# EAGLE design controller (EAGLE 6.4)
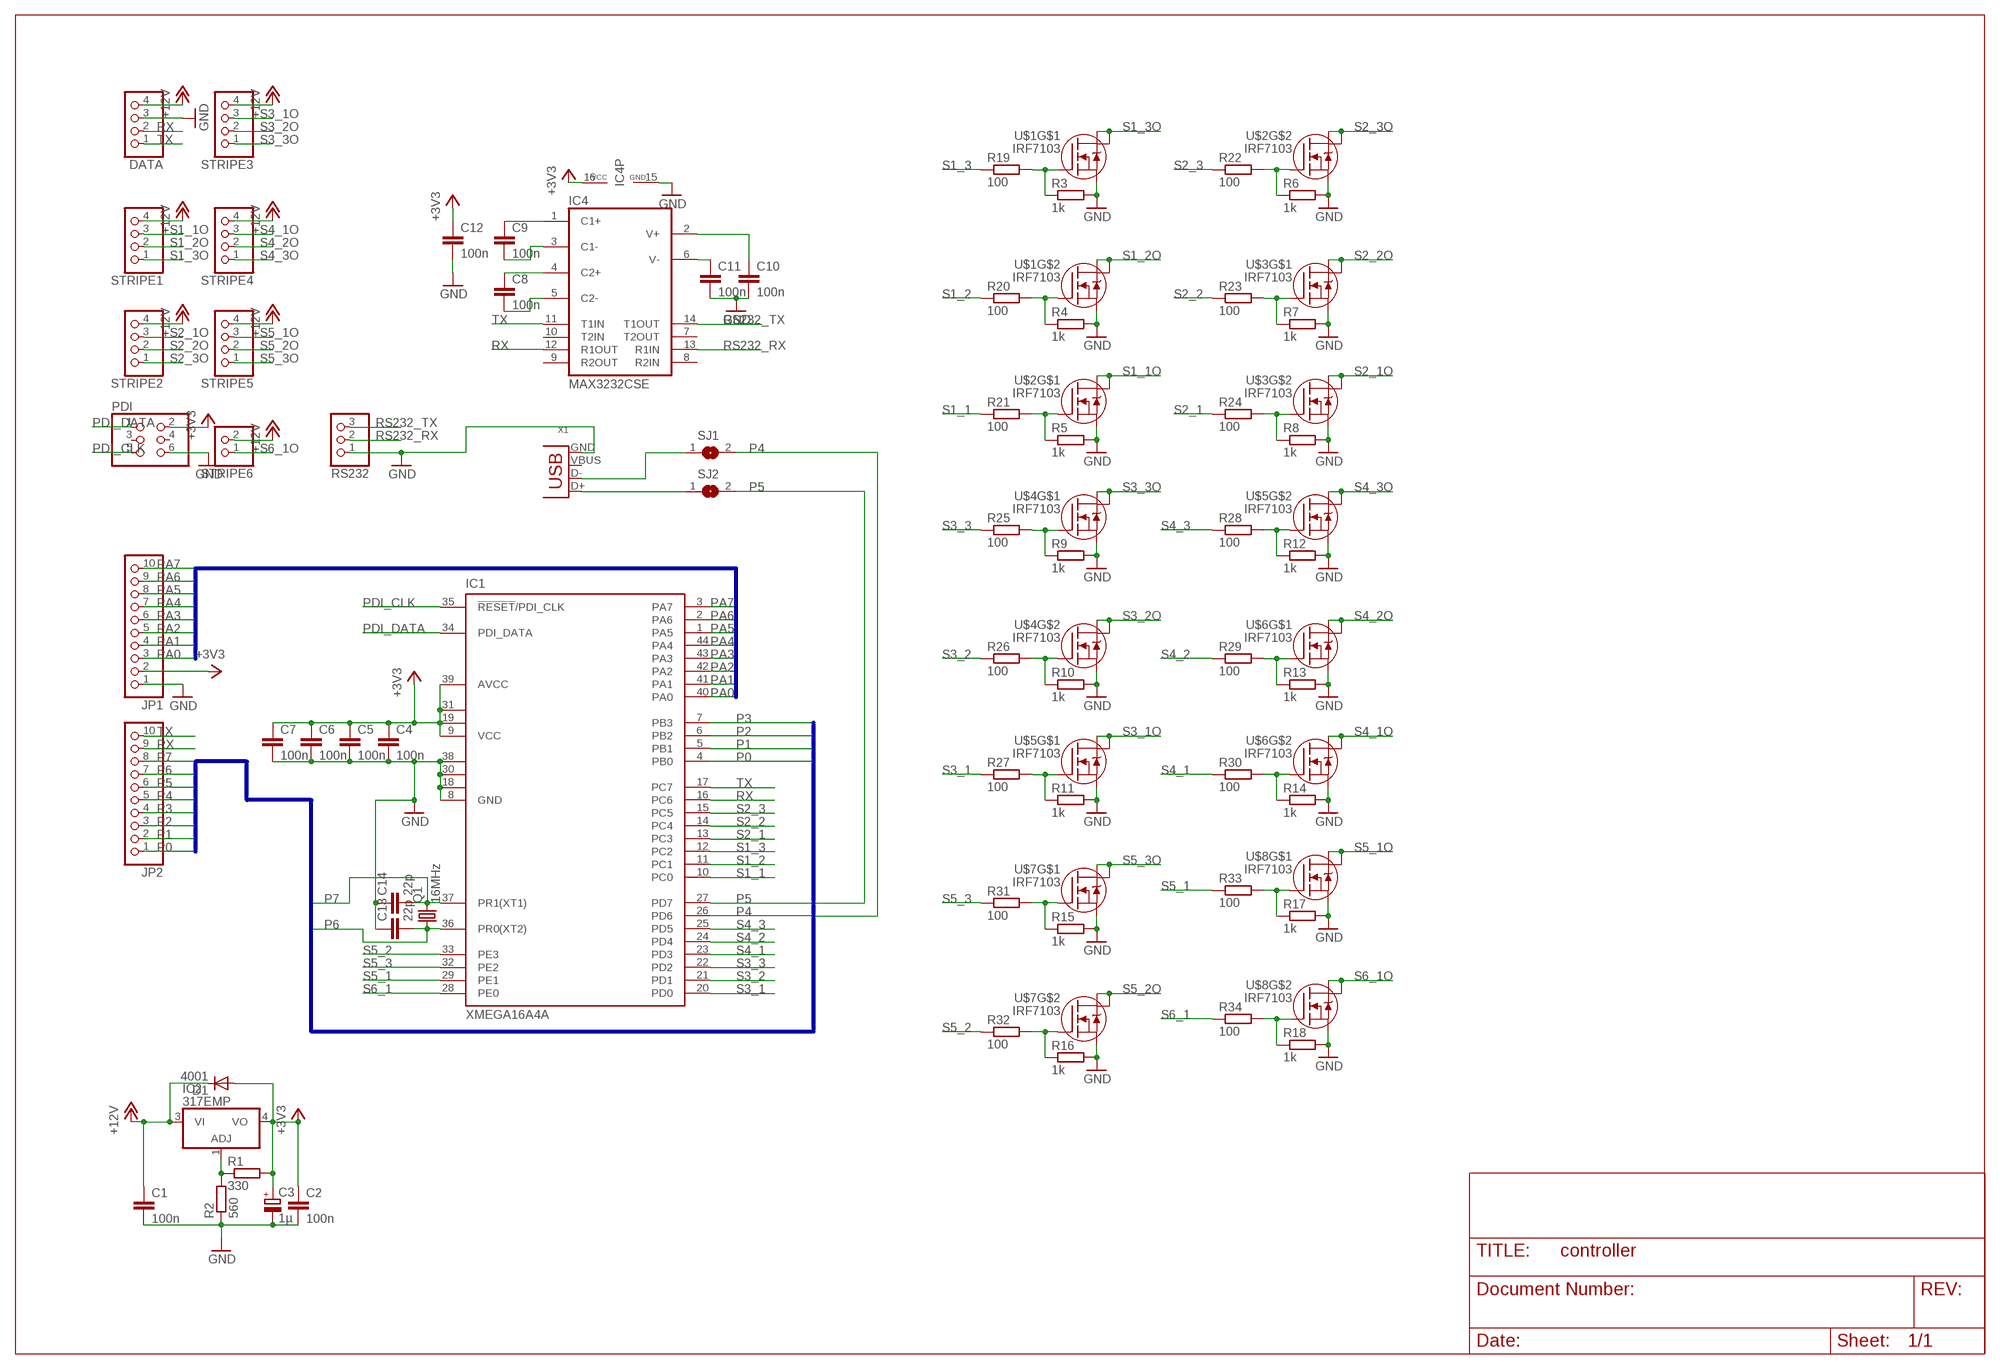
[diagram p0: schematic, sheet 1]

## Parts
C1  100n  C-EUC0805K  [C0805K]
C2  100n  C-EUC0805K  [C0805K]
C3  1µ  CPOL-EUSMCB  [SMC_B]
C4  100n  C-EUC0805K  [C0805K]
C5  100n  C-EUC0805K  [C0805K]
C6  100n  C-EUC0805K  [C0805K]
C7  100n  C-EUC0805K  [C0805K]
C8  100n  C-EUC0805K  [C0805K]
C9  100n  C-EUC0805K  [C0805K]
C10  100n  C-EUC0805K  [C0805K]
C11  100n  C-EUC0805K  [C0805K]
C12  100n  C-EUC0805K  [C0805K]
C13  22p  C-EUC0805K  [C0805K]
C14  22p  C-EUC0805K  [C0805K]
D1  4001  DIODE-MELF-MLL41  [MELF-MLL41]
DATA  PINHD-1X4  [1X04]
IC1  XMEGA16A4A  [TQFP44]
IC2  317EMP  [SOT223]
IC4  MAX3232CSE  [SO16]
JP1  PINHD-1X10  [1X10]
JP2  PINHD-1X10  [1X10]
PDI  PINHD-2X3  [2X03]
Q1  16MHz  CRYSTALHC49S  [HC49/S]
R1  330  R-EU_R0603  [R0603]
R2  560  R-EU_R0603  [R0603]
R3  1k  R-EU_R0603  [R0603]
R4  1k  R-EU_R0603  [R0603]
R5  1k  R-EU_R0603  [R0603]
R6  1k  R-EU_R0603  [R0603]
R7  1k  R-EU_R0603  [R0603]
R8  1k  R-EU_R0603  [R0603]
R9  1k  R-EU_R0603  [R0603]
R10  1k  R-EU_R0603  [R0603]
R11  1k  R-EU_R0603  [R0603]
R12  1k  R-EU_R0603  [R0603]
R13  1k  R-EU_R0603  [R0603]
R14  1k  R-EU_R0603  [R0603]
R15  1k  R-EU_R0603  [R0603]
R16  1k  R-EU_R0603  [R0603]
R17  1k  R-EU_R0603  [R0603]
R18  1k  R-EU_R0603  [R0603]
R19  100  R-EU_R0603  [R0603]
R20  100  R-EU_R0603  [R0603]
R21  100  R-EU_R0603  [R0603]
R22  100  R-EU_R0603  [R0603]
R23  100  R-EU_R0603  [R0603]
R24  100  R-EU_R0603  [R0603]
R25  100  R-EU_R0603  [R0603]
R26  100  R-EU_R0603  [R0603]
R27  100  R-EU_R0603  [R0603]
R28  100  R-EU_R0603  [R0603]
R29  100  R-EU_R0603  [R0603]
R30  100  R-EU_R0603  [R0603]
R31  100  R-EU_R0603  [R0603]
R32  100  R-EU_R0603  [R0603]
R33  100  R-EU_R0603  [R0603]
R34  100  R-EU_R0603  [R0603]
RS232  PINHD-1X3  [1X03]
SJ1  SJ  [SJ]
SJ2  SJ  [SJ]
STRIPE1  PINHD-1X4  [1X04]
STRIPE2  PINHD-1X4  [1X04]
STRIPE3  PINHD-1X4  [1X04]
STRIPE4  PINHD-1X4  [1X04]
STRIPE5  PINHD-1X4  [1X04]
STRIPE6  PINHD-1X2  [1X02]
U$1  IRF7103  [SO8-2]
U$2  IRF7103  [SO8-2]
U$3  IRF7103  [SO8-2]
U$4  IRF7103  [SO8-2]
U$5  IRF7103  [SO8-2]
U$6  IRF7103  [SO8-2]
U$7  IRF7103  [SO8-2]
U$8  IRF7103  [SO8-2]
X1  USB-MB-H  [USB-MB-H]

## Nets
+3V3: C2.1 C3.+ C4.1 C5.1 C6.1 C7.1 C12.1 D1.A IC1.9(VCC) IC1.19(VCC1) IC1.31(VCC2) IC1.39(AVCC) IC2.4(VO) IC4.16(VCC) JP1.2 PDI.2 R1.2
+12V: C1.1 D1.C DATA.4 IC2.3(VI) STRIPE1.4 STRIPE2.4 STRIPE3.4 STRIPE4.4 STRIPE5.4 STRIPE6.2
GND: C1.2 C2.2 C3.- C4.2 C5.2 C6.2 C7.2 C10.2 C11.2 C12.2 C13.1 C14.1 DATA.3 IC1.8(GND) IC1.18(GND1) IC1.30(GND2) IC1.38(GND3) IC4.15(GND) JP1.1 PDI.6 R2.1 R3.2 R4.2 R5.2 R6.2 R7.2 R8.2 R9.2 R10.2 R11.2 R12.2 R13.2 R14.2 R15.2 R16.2 R17.2 R18.2 RS232.1 U$1.1(S) U$1.3(S) U$2.1(S) U$2.3(S) U$3.1(S) U$3.3(S) U$4.1(S) U$4.3(S) U$5.1(S) U$5.3(S) U$6.1(S) U$6.3(S) U$7.1(S) U$7.3(S) U$8.1(S) U$8.3(S) X1.GND
N$1: C8.1 IC4.4(C2+)
N$2: C8.2 IC4.5(C2-)
N$3: C9.1 IC4.1(C1+)
N$4: IC2.1(ADJ) R1.1 R2.2
N$5: C9.2 IC4.3(C1-)
N$6: C10.1 IC4.2(V+)
N$7: C11.1 IC4.6(V-)
N$8: R3.1 R19.2 U$1.2(G)
N$9: R4.1 R20.2 U$1.4(G)
N$10: R5.1 R21.2 U$2.2(G)
N$11: R6.1 R22.2 U$2.4(G)
N$12: R8.1 R24.2 U$3.4(G)
N$13: R11.1 R27.2 U$5.2(G)
N$14: R7.1 R23.2 U$3.2(G)
N$15: R12.1 R28.2 U$5.4(G)
N$16: R9.1 R25.2 U$4.2(G)
N$17: R10.1 R26.2 U$4.4(G)
N$18: R14.1 R30.2 U$6.4(G)
N$19: R15.1 R31.2 U$7.2(G)
N$20: R13.1 R29.2 U$6.2(G)
N$21: R18.1 R34.2 U$8.4(G)
N$22: R16.1 R32.2 U$7.4(G)
N$23: SJ2.1 X1.D+
N$24: R17.1 R33.2 U$8.2(G)
N$25: SJ1.1 X1.D-
P0: IC1.4(PB0) JP2.1
P1: IC1.5(PB1) JP2.2
P2: IC1.6(PB2) JP2.3
P3: IC1.7(PB3) JP2.4
P4: IC1.26(PD6) JP2.5 SJ1.2
P5: IC1.27(PD7) JP2.6 SJ2.2
P6: C13.2 IC1.36(PR0(XT2)) JP2.7 Q1.1
P7: C14.2 IC1.37(PR1(XT1)) JP2.8 Q1.2
PA0: IC1.40(PA0) JP1.3
PA1: IC1.41(PA1) JP1.4
PA2: IC1.42(PA2) JP1.5
PA3: IC1.43(PA3) JP1.6
PA4: IC1.44(PA4) JP1.7
PA5: IC1.1(PA5) JP1.8
PA6: IC1.2(PA6) JP1.9
PA7: IC1.3(PA7) JP1.10
PDI_CLK: IC1.35(!RESET!/PDI_CLK) PDI.5
PDI_DATA: IC1.34(PDI_DATA) PDI.1
RS232_RX: IC4.13(R1IN) RS232.2
RS232_TX: IC4.14(T1OUT) RS232.3
RX: DATA.2 IC1.16(PC6) IC4.12(R1OUT) JP2.9
S1_1: IC1.10(PC0) R21.1
S1_1O: STRIPE1.3 U$2.7(D) U$2.8(D)
S1_2: IC1.11(PC1) R20.1
S1_2O: STRIPE1.2 U$1.5(D) U$1.6(D)
S1_3: IC1.12(PC2) R19.1
S1_3O: STRIPE1.1 U$1.7(D) U$1.8(D)
S2_1: IC1.13(PC3) R24.1
S2_1O: STRIPE2.3 U$3.5(D) U$3.6(D)
S2_2: IC1.14(PC4) R23.1
S2_2O: STRIPE2.2 U$3.7(D) U$3.8(D)
S2_3: IC1.15(PC5) R22.1
S2_3O: STRIPE2.1 U$2.5(D) U$2.6(D)
S3_1: IC1.20(PD0) R27.1
S3_1O: STRIPE3.3 U$5.7(D) U$5.8(D)
S3_2: IC1.21(PD1) R26.1
S3_2O: STRIPE3.2 U$4.5(D) U$4.6(D)
S3_3: IC1.22(PD2) R25.1
S3_3O: STRIPE3.1 U$4.7(D) U$4.8(D)
S4_1: IC1.23(PD3) R30.1
S4_1O: STRIPE4.3 U$6.5(D) U$6.6(D)
S4_2: IC1.24(PD4) R29.1
S4_2O: STRIPE4.2 U$6.7(D) U$6.8(D)
S4_3: IC1.25(PD5) R28.1
S4_3O: STRIPE4.1 U$5.5(D) U$5.6(D)
S5_1: IC1.29(PE1) R33.1
S5_1O: STRIPE5.3 U$8.7(D) U$8.8(D)
S5_2: IC1.33(PE3) R32.1
S5_2O: STRIPE5.2 U$7.5(D) U$7.6(D)
S5_3: IC1.32(PE2) R31.1
S5_3O: STRIPE5.1 U$7.7(D) U$7.8(D)
S6_1: IC1.28(PE0) R34.1
S6_1O: STRIPE6.1 U$8.5(D) U$8.6(D)
TX: DATA.1 IC1.17(PC7) IC4.11(T1IN) JP2.10
Unconnected: IC4.7(T2OUT) IC4.8(R2IN) IC4.9(R2OUT) IC4.10(T2IN) PDI.3 PDI.4 X1.VBUS

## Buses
EXP1:PA[0..7]
EXP2:P[0..7]

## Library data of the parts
C1 C2 C4-C14 = resistor:C-EU: CAPACITOR, European symbol
C3 = resistor:CPOL-EU: POLARIZED CAPACITOR, European symbol
D1 = diode:DIODE-: DIODE
DATA STRIPE1-STRIPE5 = pinhead:PINHD-1X4: PIN HEADER
IC1 = atmel:XMEGA16A4: MICROCONTROLLER Features High-performance, Low-power 8/16-bit AVR XMEGA Microcontroller Non-Volatile Program and Data Memories - 16 KB - 128 KB of In-System Self-Programmable Flash - 4 KB - 8 KB Boot Code Section with Independent Lock Bits - 1 KB - 2 KB EEPROM - 2 KB - 8 KB Internal SRAM Peripheral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; OC_FARNELL: unknown; OC_NEWARK: unknown
IC2 = linear:*317: Positive VOLTAGE REGULATOR
IC4 = maxim:MAX3232*: True RS-232 Transceivers 3.0V to 5.5V, Low-Power up to 1Mbps, Using Four 0.1µF External Capacitors Source: http://pdfserv.maxim-ic.com/en/ds/MAX3222-MAX3241.pdf; MPN: MAX3232CSE; OC_FARNELL: 9725490; OC_NEWARK: 90C2890
JP1 JP2 = pinhead:PINHD-1X10: PIN HEADER
PDI = pinhead:PINHD-2X3: PIN HEADER
Q1 = crystal:CRYSTAL: CRYSTAL; OC_FARNELL: 1667008; OC_NEWARK: unknown
R1-R34 = resistor:R-EU_: RESISTOR, European symbol
RS232 = pinhead:PINHD-1X3: PIN HEADER
SJ1 SJ2 = jumper:SJ: SMD solder JUMPER
STRIPE6 = pinhead:PINHD-1X2: PIN HEADER
U$1-U$8 = irf-2:IRF7103: HEXFET® Power MOSFET Adavanced Process Technology Ultra Low On-Resistance Dual N-Channel MOSFET Surface Mount Available in Tape & Reel Dynamic dv/dt Rating Fast Switching Please connect both Drain-Pins of each FET for thermal Reasons! (Pin 5 with Pin 6, 7 with 8)
X1 = con-usb:USB: USB Connectors

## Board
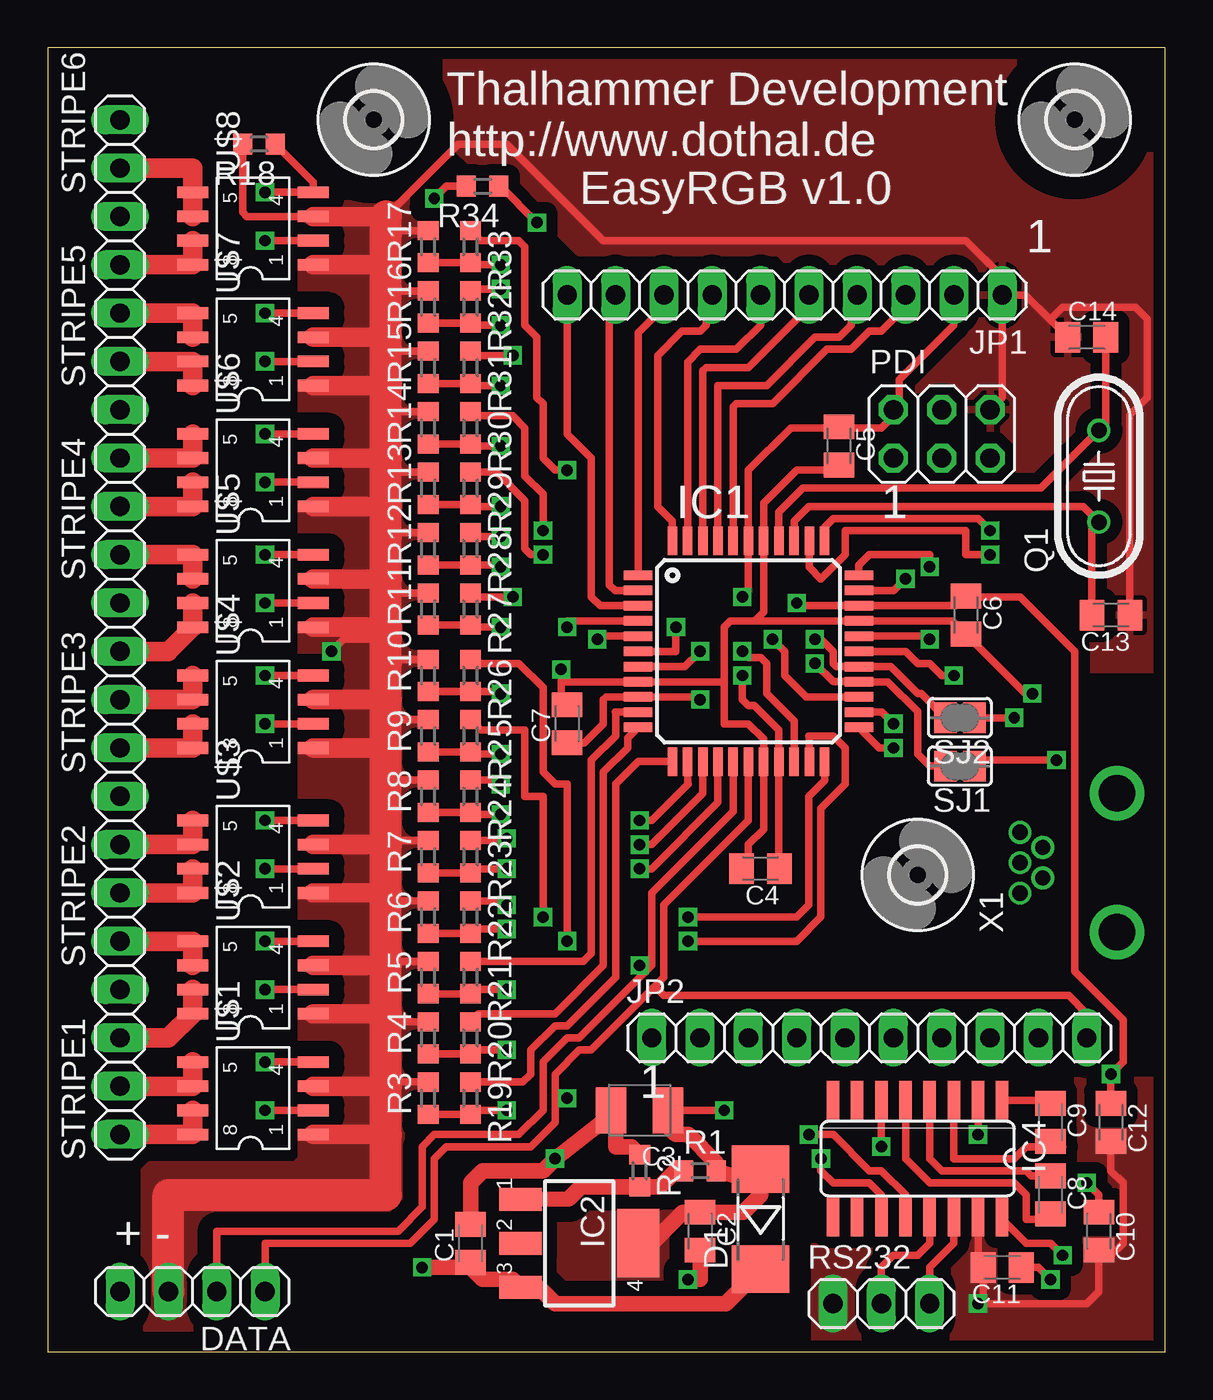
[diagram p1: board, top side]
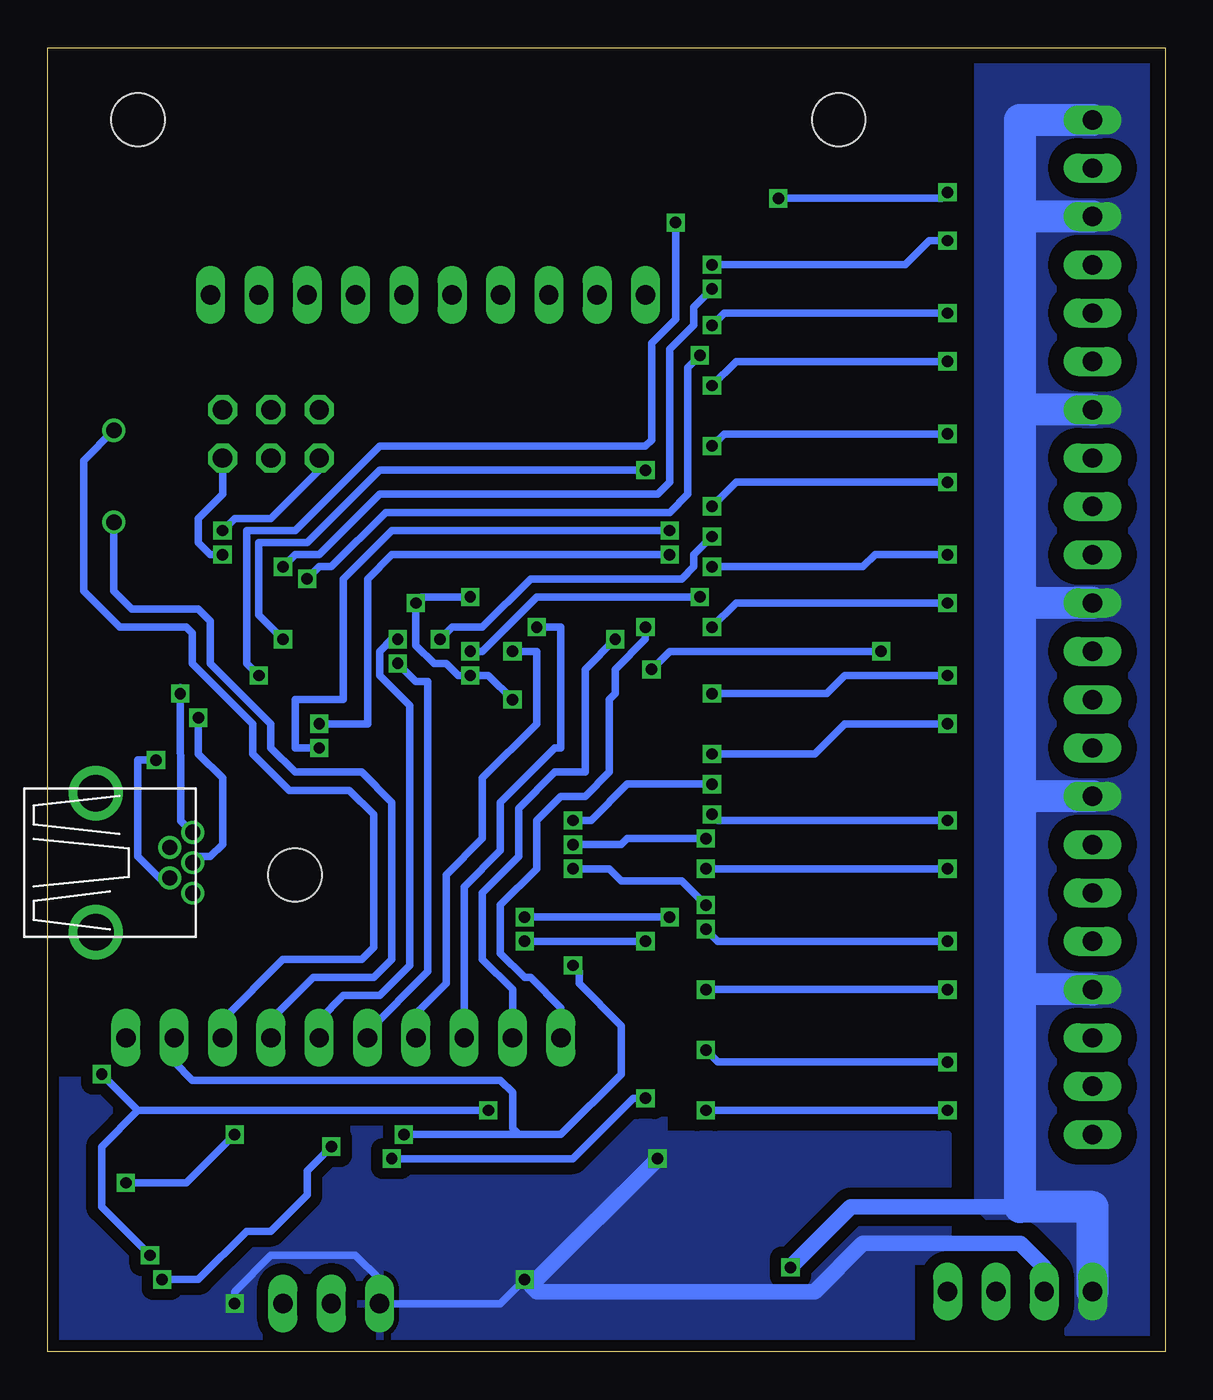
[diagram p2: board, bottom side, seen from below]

Size 58.73 x 68.57 mm. Coordinates in mm from the lower left corner, seen from the top.
Outline: 0,0 58.73,0 58.73,68.57 0,68.57 0,0
Copper layers (1*16): Top 0.0356mm / dielectric 1.5011mm / Bottom 0.0356mm
Design rules "LaenPCBOrder": minimum track width 6mil, minimum drill 13mil, track to track 6mil, track to pad 6mil, pad to pad 6mil, via to via 6mil, smd to smd 6mil, copper to edge 15mil, drill to drill 6mil, minimum pad ring 7mil, minimum via ring 7mil, stop-mask expansion 4mil, vias tented up to drill 0mil, thermal gap 10mil

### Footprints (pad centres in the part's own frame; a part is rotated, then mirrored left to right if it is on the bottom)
C0805K = smd 1.3 x 1.6: 1 -1,0; 2 1,0
SMC_B = smd 1.6 x 2.4: + -1.5,0; - 1.5,0
MELF-MLL41 = smd 2.5 x 3: A 2.625,0; C -2.625,0
1X04 = drill 1.016 long: 1 -3.81,0; 2 -1.27,0; 3 1.27,0; 4 3.81,0
TQFP44 = smd 1.5 x 0.5: 1 -5.8,4; 2 -5.8,3.2; 3 -5.8,2.4; 4 -5.8,1.6; 5 -5.8,0.8; 6 -5.8,0; 7 -5.8,-0.8; 8 -5.8,-1.6; 9 -5.8,-2.4; 10 -5.8,-3.2; 11 -5.8,-4; 23 5.8,-4; 24 5.8,-3.2; 25 5.8,-2.4; 26 5.8,-1.6; 27 5.8,-0.8; 28 5.8,0; 29 5.8,0.8; 30 5.8,1.6; 31 5.8,2.4; 32 5.8,3.2; 33 5.8,4 | smd 0.5 x 1.5: 12 -4,-5.8; 13 -3.2,-5.8; 14 -2.4,-5.8; 15 -1.6,-5.8; 16 -0.8,-5.8; 17 0,-5.8; 18 0.8,-5.8; 19 1.6,-5.8; 20 2.4,-5.8; 21 3.2,-5.8; 22 4,-5.8; 34 4,5.8; 35 3.2,5.8; 36 2.4,5.8; 37 1.6,5.8; 38 0.8,5.8; 39 0,5.8; 40 -0.8,5.8; 41 -1.6,5.8; 42 -2.4,5.8; 43 -3.2,5.8; 44 -4,5.8
SOT223 = smd 1.219 x 2.235: 1 -2.311,-3.099; 2 0,-3.099; 3 2.311,-3.099 | smd 3.6 x 2.2: 4 0,3.099
SO16 = smd 0.66 x 2.032: 1 -4.445,-3.073; 2 -3.175,-3.073; 3 -1.905,-3.073; 4 -0.635,-3.073; 5 0.635,-3.073; 6 1.905,-3.073; 7 3.175,-3.073; 8 4.445,-3.073; 9 4.445,3.073; 10 3.175,3.073; 11 1.905,3.073; 12 0.635,3.073; 13 -0.635,3.073; 14 -1.905,3.073; 15 -3.175,3.073; 16 -4.445,3.073
1X10 = drill 1.016 long: 1 -11.43,0; 2 -8.89,0; 3 -6.35,0; 4 -3.81,0; 5 -1.27,0; 6 1.27,0; 7 3.81,0; 8 6.35,0; 9 8.89,0; 10 11.43,0
2X03 = drill 1.016 octagon: 1 -2.54,-1.27; 2 -2.54,1.27; 3 0,-1.27; 4 0,1.27; 5 2.54,-1.27; 6 2.54,1.27
HC49/S = drill 0.813: 1 -2.413,0; 2 2.413,0
R0603 = smd 1 x 1.1: 1 -0.85,0; 2 0.85,0
1X03 = drill 1.016 long: 1 -2.54,0; 2 0,0; 3 2.54,0
SJ = smd 1.168 x 1.6: 1 -0.762,0; 2 0.762,0
1X02 = drill 1.016 long: 1 -1.27,0; 2 1.27,0
SO8-2 = smd 0.61 x 1.626: 1 -2.54,-2.54; 2 -1.27,-2.54; 3 0,-2.54; 4 1.27,-2.54; 5 1.27,3.81; 6 0,3.81; 7 -1.27,3.81; 8 -2.54,3.81
2,8 = hole 2.8: 0,0
USB-MB-H = drill 0.8: D+ 5.1,0; D- 3.9,0.8; GND 5.1,-1.6; ID 3.9,-0.8; VBUS 5.1,1.6 | drill 1.9: P$6 0,-3.65; P$7 0,3.65

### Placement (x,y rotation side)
C1  22.23,5.71 90 top
C2  34.29,6.35 270 top
C3  31.11,12.7 180 top
C4  37.47,25.4 180 top
C5  41.59,47.62 270 top
C6  48.26,38.73 270 top
C7  27.3,33.02 90 top
C8  52.7,8.26 270 top
C9  52.7,12.06 270 top
C10  55.24,6.35 270 top
C11  50.16,4.45 180 top
C12  55.88,12.06 270 top
C13  55.88,38.73 180 top
C14  54.61,53.34 0 top
D1  37.47,6.99 90 top
DATA  7.62,3.17 180 top
IC1  36.83,36.83 0 top
IC2  27.94,5.71 270 top
IC4  45.72,10.16 180 top
JP1  38.73,55.56 180 top
JP2  43.18,16.51 0 top
PDI  46.99,48.26 0 top
Q1  55.24,46.04 90 top
R1  34.29,9.53 0 top
R2  31.11,9.53 270 top
R3  20,13.34 90 top
R4  20,16.51 90 top
R5  20,19.68 90 top
R6  20,22.86 90 top
R7  20,26.04 90 top
R8  20,29.21 90 top
R9  20,32.38 90 top
R10  20,35.56 90 top
R11  20,39.05 90 top
R12  20,42.23 90 top
R13  20,45.4 90 top
R14  20,48.58 90 top
R15  20,51.75 90 top
R16  20,54.93 90 top
R17  20,58.1 90 top
R18  11.11,63.5 180 top
R19  22.23,13.34 270 top
R20  22.23,16.51 270 top
R21  22.23,19.68 270 top
R22  22.23,22.86 270 top
R23  22.23,26.04 270 top
R24  22.23,29.21 270 top
R25  22.23,32.38 270 top
R26  22.23,35.56 270 top
R27  22.23,39.05 270 top
R28  22.23,42.23 270 top
R29  22.23,45.4 270 top
R30  22.23,48.58 270 top
R31  22.23,51.75 270 top
R32  22.23,54.93 270 top
R33  22.23,58.1 270 top
R34  22.86,61.28 180 top
RS232  43.81,2.54 0 top
SJ1  47.94,30.8 180 top
SJ2  47.94,33.34 180 top
STRIPE1  3.81,15.24 90 top
STRIPE2  3.81,25.4 90 top
STRIPE3  3.81,35.56 90 top
STRIPE4  3.81,45.72 90 top
STRIPE5  3.81,55.88 90 top
STRIPE6  3.81,63.5 90 top
U$1  11.43,13.97 90 top
U$2  11.43,20.32 90 top
U$3  11.43,26.67 90 top
U$4  11.43,34.29 90 top
U$5  11.43,40.64 90 top
U$6  11.43,46.99 90 top
U$7  11.43,53.34 90 top
U$8  11.43,59.69 90 top
U$9  [2,8]  45.72,25.08 0 top
U$10  [2,8]  17.14,64.77 0 top
U$11  [2,8]  53.98,64.77 0 top
X1  56.2,25.72 180 top

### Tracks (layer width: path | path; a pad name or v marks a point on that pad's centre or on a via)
+3V3  (via drill 0.6)
  Top 0.406: v39.37,39.37 39.51,39.23 IC1.31 47.76,39.23 C6.1 48.62,39.37 48.94,39.69 51.12,39.69 53.98,36.83 53.98,20 56.52,17.46 56.52,15.24 v55.88,14.61 C12.1 | v34.29,34.29 34.15,34.43 IC1.9 29.35,34.43 29.21,34.29 29.21,33.02 28.21,32.02 C7.1 | C4.1 38.43,25.43 IC1.19 38.43,32.69 37.15,33.97 36.83,33.97 36.51,34.29 v36.51,35.56 | C3.+ v35.56,12.7 | IC4.16 50.16,6.99 51.44,5.71 52.7,5.71 v53.34,5.08 | v36.51,39.69 36.83,40.01 IC1.39 36.83,46.35 39.05,48.58 41.55,48.58 C5.1 41.64,48.58 43.81,48.58 44.45,49.21 PDI.2 44.77,49.85 44.77,51.12 47.62,53.98 JP1.2
  Top 0.813: IC2.4 31.11,5.08 33.38,7.35 C2.1 36.56,7.35 37.47,8.26 D1.A 37.38,8.89 R1.2 35.14,9.95 33.66,11.43 33.02,11.43 32.38,12.06 32.38,12.47 C3.+
  Bottom 0.406: v34.29,34.29 35.56,35.56 v36.51,35.56 37.15,35.56 37.78,36.2 38.42,36.2 39.37,37.15 v39.37,39.37 39.05,39.69 v36.51,39.69 | 53.98,12.7 v55.88,14.61 | v35.56,12.7 53.98,12.7 | v53.34,5.08 55.88,7.62 55.88,10.79 53.98,12.7
  pour Top (isolate 0.813, no thermals): 26.67,7.3 32.7,7.3 32.7,3.81 26.67,3.81
+12V  (via drill 0.6)
  Top 0.813: 37.55,4.45 D1.C 35.65,2.54 26.67,2.54 25.81,3.4 IC2.3 24.43,3.81 22.86,3.81 22.23,4.45 C1.1 21.95,4.45 v19.68,4.45
  Bottom 0.813: 7.62,7.62 16.51,7.62 v19.68,4.45
  Bottom 1.676: DATA.4 3.81,7.62 7.62,7.62 7.62,19.05 | 7.62,19.05 7.62,29.21 | 7.62,29.21 7.62,39.37 | 7.62,39.37 7.62,49.53 | 7.62,49.53 7.62,59.69 | 7.62,59.69 7.62,64.77 STRIPE6.2 | STRIPE5.4 7.62,59.69 | STRIPE4.4 7.62,49.53 | STRIPE3.4 7.62,39.37 | STRIPE2.4 7.62,29.21 | STRIPE1.4 7.62,19.05
  pour Bottom (isolate 0.813, no thermals): 0,0.95 5.08,0.95 5.08,4.45 6.99,6.35 8.57,6.35 9.84,7.62 9.84,68.58 0,68.58
GND  (via drill 0.6)
  Top 0.406: 35.56,35.23 IC1.8 27,35.23 | 37.16,38.43 IC1.30 47.56,38.43 C6.2 | 37.16,38.43 37.63,38.9 IC1.38 37.63,44.62 39.37,46.35 41.32,46.35 C5.2 | 17.78,59.69 21.59,63.5 24.13,63.5 29.21,58.42 48.26,58.42 50.16,56.52 JP1.1 | 35.56,35.23 35.56,33.02 36.83,33.02 37.63,32.22 IC1.18 37.63,27.47 36.83,26.67 36.83,25.77 C4.2 | 47.9,37.47 C6.2 | 27,35.23 27,34.33 C7.2 | IC4.15 48.9,4.71 C11.2 49.16,2.81 v48.9,2.54 54.61,2.54 55.24,3.17 C10.2 55.52,5.08 55.88,5.08 56.52,5.71 56.52,8.89 55.88,9.53 C12.2 | R3.2 18,14.19 17.78,13.97 | R4.2 18,17.36 17.78,17.14 | R6.2 18,23.71 17.78,23.5 | R5.2 18.2,20.54 17.78,20.95 | R7.2 18,26.89 17.78,26.67 | R8.2 17.88,30.06 17.78,30.16 | 17.78,37.47 15.56,37.47 v14.92,36.83 | v26.99,35.88 26.99,35.24 27,35.23 | R10.2 18,36.41 17.78,36.2 | R9.2 17.88,33.23 17.78,33.34 | R11.2 17.88,39.9 17.78,40.01 | R12.2 18,43.08 17.78,42.86 | 35.56,35.23 35.56,38.1 35.88,38.42 37.15,38.42 37.16,38.43 | R14.2 17.88,49.43 17.78,49.53 | R13.2 17.88,46.25 17.78,46.35 | R15.2 17.88,52.6 17.78,52.7 | R16.2 17.88,55.78 17.78,55.88 | R17.2 18,58.95 17.78,58.74 | R18.2 10.26,59.91 10.48,59.69 U$8.3 | v51.75,34.61 51.39,34.61 C6.2 | JP1.1 50.16,50.16 PDI.6 | JP1.1 51.39,55.56 52.68,54.27 | 52.68,54.27 C14.1 | C13.1 56.88,49.26 57.78,50.16 57.78,54.29 57.15,54.93 53.34,54.93 52.68,54.27
  Top 0.813: C2.2 34.29,3.81 v33.66,3.81 | R2.1 30.7,10.79 29.84,10.79 29.84,12.47 C3.- 29.61,12.47 v26.67,10.16 26.04,9.53 22.86,9.53 22.23,8.89 C1.2
  Top 1.016: 17.78,59.69 U$8.3 | U$8.1 17.78,57.15 | U$7.3 17.78,53.34 | U$7.1 17.78,50.8 | U$6.3 17.78,46.99 | U$6.1 17.78,44.45 | U$5.3 17.78,40.64 | U$5.1 17.78,38.1 | U$4.3 17.78,34.29 | U$4.1 17.78,31.75 | U$3.3 17.78,26.67 | U$3.1 17.78,24.13 | U$2.3 17.78,20.32 | U$2.1 17.78,17.78 | U$1.3 17.78,13.97 | U$1.1 17.78,11.43
  Top 1.676: DATA.3 6.35,8.26 17.78,8.26 17.78,11.43 17.78,13.97 17.78,17.14 17.78,17.78 17.78,20.32 17.78,20.95 17.78,23.5 17.78,24.13 17.78,26.67 17.78,30.16 17.78,31.75 17.78,33.34 17.78,34.29 17.78,36.2 17.78,37.47 17.78,38.1 17.78,40.01 17.78,40.64 17.78,42.86 17.78,44.45 17.78,46.35 17.78,46.99 17.78,49.53 17.78,50.8 17.78,52.7 17.78,53.34 17.78,55.88 17.78,57.15 17.78,58.74 17.78,59.69
  Bottom 0.406: v33.66,3.81 34.92,2.54 RS232.1 41.27,3.81 42.55,5.08 46.99,5.08 48.9,3.17 v48.9,2.54 | v14.92,36.83 26.04,36.83 v26.99,35.88 | X1.GND 51.73,27.92 51.75,34.92 v51.75,34.61
  Bottom 0.813: DATA.3 6.35,4.45 7.62,5.71 15.88,5.71 18.41,3.17 33.02,3.17 v33.66,3.81 33.02,3.81 v26.67,10.16
  pour Top (isolate 0.61): 20.95,68.58 20.95,63.82 22.86,61.91 23.81,61.91 27.94,57.78 38.42,57.78 48.26,47.94 48.26,40.01 52.39,35.88 58.74,35.88 59.05,68.26 58.74,68.58
  pour Top (isolate 0.813, no thermals): 13.34,61.91 19.37,61.91 19.37,7.94 18.1,6.67 7.94,6.67 7.94,1.27 5.08,1.27 5.08,9.53 5.4,9.84 13.02,9.84 13.34,10.16
  pour Top (isolate 0.61, no thermals): 40.32,13.97 40.32,0.64 58.1,0.64 58.1,14.29 40.32,14.29
  pour Bottom (isolate 0.61): 26.35,15.24 26.35,11.43 11.43,11.43 11.43,4.76 13.34,4.76 13.34,0.64 58.1,0.64 58.1,14.29 30.48,14.29 30.48,15.24
N$1
  Top 0.406: C8.1 51.7,9.26 51.44,9.53 46.99,9.53 46.35,10.16 IC4.4
N$2
  Top 0.406: IC4.5 45.09,10.16 46.35,8.89 50.8,8.89 51.44,8.26 51.44,6.99 52.44,6.99 C8.2
N$3
  Top 0.406: IC4.1 52.54,13.23 C9.1
N$4
  Top 0.813: IC2.1 27.39,8.04 28.03,8.68 R2.2 32.17,8.68 33.02,9.53 R1.1
N$5
  Top 0.406: IC4.3 47.62,10.16 50.8,10.16 51.44,10.79 52.98,10.79 | 53.34,10.79 52.98,10.79 | 52.98,10.79 C9.2
N$6  (via drill 0.6)
  Top 0.406: C10.1 55.24,8.26 v54.61,8.89 | v48.9,11.43 IC4.2
  Bottom 0.406: v54.61,8.89 51.44,8.89 v48.9,11.43
N$7  (via drill 0.6)
  Top 0.406: v43.81,10.79 IC4.6 | C11.1 52.07,4.45 v52.7,3.81
  Bottom 0.406: v43.81,10.79 45.09,9.53 45.09,8.26 46.99,6.35 48.26,6.35 50.8,3.81 v52.7,3.81
N$8  (via drill 0.6)
  Top 0.406: R3.1 R19.2 22.44,12.7 v24.13,12.7 | U$1.2 v11.43,12.7
  Bottom 0.406: v11.43,12.7 v24.13,12.7
N$9  (via drill 0.6)
  Top 0.406: R4.1 R20.2 22.44,15.88 v24.13,15.88 | U$1.4 v11.43,15.24
  Bottom 0.406: v11.43,15.24 23.5,15.24 v24.13,15.88
N$10  (via drill 0.6)
  Top 0.406: R5.1 R21.2 22.44,19.05 v24.13,19.05 | U$2.2 v11.43,19.05
  Bottom 0.406: v11.43,19.05 v24.13,19.05
N$11  (via drill 0.6)
  Top 0.406: R6.1 R22.2 22.44,22.23 v24.13,22.23 | U$2.4 v11.43,21.59
  Bottom 0.406: v11.43,21.59 23.5,21.59 v24.13,22.23
N$12  (via drill 0.6)
  Top 0.406: R8.1 R24.2 22.33,28.26 v23.81,28.26 | U$3.4 v11.43,27.94
  Bottom 0.406: v11.43,27.94 23.5,27.94 v23.81,28.26
N$13  (via drill 0.6)
  Top 0.406: U$5.2 v11.43,39.37 | v23.81,38.1 22.33,38.1 R27.2 R11.1
  Bottom 0.406: v11.43,39.37 22.54,39.37 v23.81,38.1
N$14  (via drill 0.6)
  Top 0.406: R7.1 R23.2 22.44,25.4 v24.13,25.4 | U$3.2 v11.43,25.4
  Bottom 0.406: v11.43,25.4 v24.13,25.4
N$15  (via drill 0.6)
  Top 0.406: R12.1 R28.2 23.71,41.38 v23.81,41.27 | v11.43,41.91 U$5.4
  Bottom 0.406: v23.81,41.27 15.88,41.27 15.24,41.91 v11.43,41.91
N$16  (via drill 0.6)
  Top 0.406: U$4.2 v11.43,33.02 | v23.81,31.43 22.33,31.43 R25.2 R9.1
  Bottom 0.406: v11.43,33.02 16.83,33.02 18.41,31.43 v23.81,31.43
N$17  (via drill 0.6)
  Top 0.406: R10.1 R26.2 23.71,34.71 v23.81,34.61 | v11.43,35.56 U$4.4
  Bottom 0.406: v23.81,34.61 17.78,34.61 16.83,35.56 v11.43,35.56
N$18  (via drill 0.6)
  Top 0.406: R14.1 R30.2 22.33,47.62 v23.81,47.62 | U$6.4 v11.43,48.26
  Bottom 0.406: v11.43,48.26 23.18,48.26 v23.81,47.62
N$19  (via drill 0.6)
  Top 0.406: R15.1 R31.2 22.33,50.8 v23.81,50.8 | U$7.2 v11.43,52.07
  Bottom 0.406: v11.43,52.07 22.54,52.07 v23.81,50.8
N$20  (via drill 0.6)
  Top 0.406: R13.1 R29.2 22.33,44.45 v23.81,44.45 | U$6.2 v11.43,45.72
  Bottom 0.406: v11.43,45.72 22.54,45.72 v23.81,44.45
N$21  (via drill 0.6)
  Top 0.406: R34.2 20.95,61.28 v20.32,60.64 | v11.43,60.96 U$8.4 13.97,61.49 R18.1
  Bottom 0.406: v20.32,60.64 11.75,60.64 v11.43,60.96
N$22  (via drill 0.6)
  Top 0.406: R16.1 R32.2 22.33,53.98 v23.81,53.98 | U$7.4 v11.43,54.61
  Bottom 0.406: v11.43,54.61 23.18,54.61 v23.81,53.98
N$23  (via drill 0.6)
  Top 0.406: SJ2.1 v50.8,33.34
  Bottom 0.406: v50.8,33.34 50.8,31.43 49.53,30.16 49.53,26.67 50.16,26.04 50.78,26.04 X1.D+
N$24  (via drill 0.6)
  Top 0.406: R17.1 R33.2 22.33,57.15 v23.81,57.15 | U$8.2 v11.43,58.42
  Bottom 0.406: v11.43,58.42 12.38,58.42 13.65,57.15 v23.81,57.15
N$25  (via drill 0.6)
  Top 0.406: v53.02,31.11 49.02,31.11 SJ1.1
  Bottom 0.406: X1.D- 52.86,24.92 53.98,26.04 53.98,31.11 v53.02,31.11
P0  (via drill 0.6)
  Top 0.406: IC1.4 27.32,38.43 v27.3,38.1
  Bottom 0.406: v27.3,38.1 27.3,37.47 28.89,35.88 28.89,34.61 29.21,34.29 29.21,30.48 30.48,29.21 31.75,29.21 33.02,27.94 33.02,25.4 34.92,23.5 34.92,20.95 33.66,19.68 33.34,19.68 31.75,18.1 JP2.1
P1  (via drill 0.6)
  Top 0.406: IC1.5 29.06,37.63 v28.89,37.47
  Bottom 0.406: v28.89,37.47 30.48,35.88 30.48,30.48 32.07,30.48 33.97,28.57 33.97,26.04 35.88,24.13 35.88,20.64 34.29,19.05 JP2.2
P2  (via drill 0.6)
  Top 0.406: v33.02,38.1 33.02,36.83 IC1.6
  Bottom 0.406: v33.02,38.1 31.75,38.1 31.75,31.75 32.07,31.75 34.92,28.89 34.92,26.35 36.83,24.45 JP2.3
P3  (via drill 0.6)
  Top 0.406: IC1.7 33.49,36.03 v34.29,36.83
  Bottom 0.406: v34.29,36.83 33.02,36.83 33.02,33.02 35.88,30.16 35.88,26.99 37.78,25.08 37.78,19.37 39.37,17.78 JP2.4
P4  (via drill 0.6)
  Top 0.406: v40.32,36.2 41.27,35.24 42.62,35.24 IC1.26 44.15,35.23 45.72,33.66 45.72,31.43 46.35,30.8 SJ1.2
  Bottom 0.406: JP2.5 41.91,16.83 38.73,20 38.73,35.24 39.37,35.24 v40.32,36.2
P5  (via drill 0.6)
  Top 0.406: v40.32,37.47 40.64,37.47 41.27,36.83 41.27,36.2 41.44,36.03 IC1.27 44.3,36.03 45.72,34.61 45.91,34.61 SJ2.2
  Bottom 0.406: v40.32,37.47 40.64,37.47 41.27,36.83 41.27,35.56 39.69,33.97 39.69,20.32 41.27,18.73 43.18,18.73 44.45,17.46 JP2.6
P6
  Top 0.406: IC1.36 39.23,43.67 40.01,44.45 54.42,44.45 Q1.1 54.88,43.26 C13.2
  Bottom 0.406: JP2.7 46.99,17.46 44.77,19.68 41.59,19.68 40.64,20.64 40.64,28.89 42.23,30.48 45.72,30.48 46.99,31.75 46.99,33.02 50.16,36.2 50.16,38.42 50.8,39.05 54.29,39.05 55.24,40.01 Q1.1
P7
  Top 0.406: IC1.37 38.43,44.15 39.69,45.4 52.2,45.4 Q1.2 55.61,48.82 C14.2
  Bottom 0.406: JP2.8 49.53,17.46 46.35,20.64 42.23,20.64 41.59,21.27 41.59,28.26 42.86,29.53 46.04,29.53 47.94,31.43 47.94,33.02 51.12,36.2 51.12,37.78 51.44,38.1 54.93,38.1 56.83,40.01 56.83,46.86 Q1.2
PA0
  Top 0.406: JP1.3 45.09,54.93 43.81,53.66 43.18,53.66 42.23,52.7 40.96,52.7 38.1,49.85 36.2,49.85 36.03,49.68 IC1.40
PA1
  Top 0.406: IC1.41 35.23,50.79 35.24,50.8 37.78,50.8 40.32,53.34 41.59,53.34 42.23,53.98 42.23,55.24 JP1.4
PA2
  Top 0.406: IC1.42 34.43,51.58 34.61,51.75 36.83,51.75 39.69,54.61 39.69,55.24 JP1.5
PA3
  Top 0.406: IC1.43 33.63,52.05 34.29,52.7 36.2,52.7 37.47,53.98 JP1.6
PA4
  Top 0.406: IC1.44 32.83,43.69 32.07,44.45 32.07,52.39 33.34,53.66 34.29,53.66 34.61,53.98 34.61,55.24 JP1.7
PA5
  Top 0.406: IC1.1 31.03,53.57 32.07,54.61 32.07,55.24 JP1.8
PA6
  Top 0.406: IC1.2 29.82,40.03 29.53,40.32 29.53,55.24 JP1.9
PA7
  Top 0.406: JP1.10 27.3,48.26 28.57,46.99 28.57,39.69 29.03,39.23 IC1.3
PDI_CLK  (via drill 0.6)
  Top 0.406: IC1.35 40.03,41.25 40.64,40.64 41.91,41.91 41.91,43.18 48.26,43.18 48.26,41.91 v49.53,41.91
  Bottom 0.406: PDI.5 49.53,45.09 50.8,43.81 50.8,42.55 50.16,41.91 v49.53,41.91
PDI_DATA  (via drill 0.6)
  Top 0.406: IC1.34 40.83,43.37 41.27,43.81 48.9,43.81 v49.53,43.18
  Bottom 0.406: PDI.1 44.45,46.35 46.99,43.81 48.9,43.81 v49.53,43.18
RS232_RX
  Top 0.406: IC4.13 46.35,5.71 45.72,5.08 44.45,5.08 43.81,4.45 RS232.2
RS232_TX
  Top 0.406: IC4.14 47.62,5.71 46.35,4.45 RS232.3
RX  (via drill 0.6)
  Top 0.406: IC1.16 36.03,28.41 31.75,24.13 31.75,20.32 31.43,20 | DATA.2 8.89,6.35 18.41,6.35 19.68,7.62 19.68,10.79 20.32,11.43 24.77,11.43 26.04,12.7 26.04,15.24 27.3,16.51 27.94,16.51 31.43,20 | IC4.12 45.09,8.26 43.81,9.53 43.18,9.53 41.27,11.43 v40.01,11.43 | v31.11,20.32 31.43,20
  Bottom 0.406: 33.97,11.43 31.75,11.43 28.57,14.61 28.57,17.14 30.8,19.37 30.8,20 v31.11,20.32 | JP2.9 52.07,15.24 51.12,14.29 34.92,14.29 34.29,13.65 34.29,11.75 33.97,11.43 | v40.01,11.43 33.97,11.43
S1_1
  Top 0.406: IC1.10 29.82,33.63 29.84,33.6 29.84,32.38 28.57,31.11 28.57,20.95 28.16,20.54 R21.1
S1_1O
  Top 1.016: U$2.7 U$2.8 6.35,16.51 STRIPE1.3
S1_2
  Top 0.406: IC1.11 30.48,32.28 30.48,31.75 29.21,30.48 29.21,20.32 26.67,17.78 22.64,17.78 R20.1
S1_2O
  Top 1.016: U$1.5 U$1.6 STRIPE1.2
S1_3
  Top 0.406: IC1.12 31.03,31.03 29.84,29.84 29.84,19.68 27.3,17.14 26.67,17.14 25.4,15.88 25.4,14.61 24.98,14.19 R19.1
S1_3O
  Top 1.016: U$1.7 U$1.8 STRIPE1.1
S2_1  (via drill 0.6)
  Top 0.406: IC1.13 33.63,29.87 33.66,29.84 31.75,27.94 v31.11,27.94 | R24.1 23.6,30.06 v23.81,29.84
  Bottom 0.406: v23.81,29.84 28.26,29.84 30.16,27.94 v31.11,27.94
S2_1O
  Top 1.016: U$3.5 U$3.6 STRIPE2.3
S2_2  (via drill 0.6)
  Top 0.406: IC1.14 34.43,29.35 31.75,26.67 v31.11,26.67 | R23.1 24.03,26.89 v24.13,26.99
  Bottom 0.406: v31.11,26.67 28.57,26.67 28.26,26.99 v24.13,26.99
S2_2O
  Top 1.016: U$3.7 U$3.8 STRIPE2.2
S2_3  (via drill 0.6)
  Top 0.406: IC1.15 35.23,28.88 31.75,25.4 v31.11,25.4 | R22.1 23.91,23.71 v24.13,23.5
  Bottom 0.406: v31.11,25.4 29.21,25.4 28.57,24.77 25.4,24.77 24.77,24.13 v24.13,23.5
S2_3O
  Top 1.016: U$2.6 U$2.5 STRIPE2.1
S3_1  (via drill 0.6)
  Top 0.406: IC1.20 39.23,33.16 37.78,34.61 37.78,36.2 37.47,36.51 36.83,36.51 v36.51,36.83 | v24.45,39.69 22.44,39.69 R27.1
  Bottom 0.406: v36.51,36.83 35.88,36.83 33.02,39.69 v24.45,39.69
S3_1O
  Top 1.016: U$5.7 U$5.8 6.35,36.83 STRIPE3.3
S3_2  (via drill 0.6)
  Top 0.406: v33.66,21.59 39.37,21.59 40.64,22.86 40.64,28.57 41.91,29.84 41.91,31.75 41.27,32.38 40.01,32.38 40.03,32.36 IC1.21 | v27.3,21.59 27.3,29.84 26.67,29.84 26.04,30.48 26.04,34.92 24.77,36.2 22.44,36.2 R26.1
  Bottom 0.406: v33.66,21.59 v27.3,21.59
S3_2O
  Top 1.016: U$4.5 U$4.6 STRIPE3.2
S3_3  (via drill 0.6)
  Top 0.406: v33.66,22.86 39.37,22.86 40.01,23.5 40.01,29.21 40.83,30.04 IC1.22 | v26.04,22.86 26.04,29.21 25.08,29.21 25.08,32.7 22.76,32.7 R25.1
  Bottom 0.406: v26.04,22.86 v33.66,22.86
S3_3O
  Top 1.016: U$4.7 U$4.8 STRIPE3.1
S4_1  (via drill 0.6)
  Top 0.406: v44.45,31.75 43.71,31.75 IC1.23 | 22.33,49.53 R30.1 22.44,49.21 24.45,49.21 25.08,48.58 25.08,46.04 26.04,45.09 v26.04,43.18
  Bottom 0.406: v44.45,31.75 45.72,31.75 45.72,34.29 43.18,34.29 43.18,40.64 40.64,43.18 v26.04,43.18
S4_1O
  Top 1.016: U$6.5 U$6.6 STRIPE4.3
S4_2  (via drill 0.6)
  Top 0.406: IC1.24 43.84,33.63 v44.45,33.02 | R29.1 23.6,46.25 25.08,44.77 25.08,42.23 25.4,41.91 v26.04,41.91
  Bottom 0.406: v26.04,41.91 40.64,41.91 41.91,40.64 41.91,33.02 v44.45,33.02
S4_2O
  Top 1.016: U$6.7 U$6.8 STRIPE4.2
S4_3  (via drill 0.6)
  Top 0.406: v23.81,42.86 22.44,42.86 R28.1 | IC1.25 39.87,34.43 38.73,35.56 38.73,36.83 v38.1,37.47
  Bottom 0.406: v38.1,37.47 37.47,38.1 35.88,38.1 33.34,40.64 25.4,40.64 24.77,41.27 24.77,41.91 v23.81,42.86
S4_3O
  Top 1.016: U$5.6 U$5.5 STRIPE4.1
S5_1  (via drill 0.6)
  Top 0.406: IC1.29 46.19,37.63 v46.35,37.47 | R33.1 22.76,58.42 24.77,58.42 25.08,58.1 25.08,53.98 25.72,53.34 25.72,50.16 26.04,49.85 26.04,46.99 26.67,46.35 v27.3,46.35
  Bottom 0.406: v46.35,37.47 47.62,38.73 47.62,42.55 45.09,42.55 41.27,46.35 v27.3,46.35
S5_1O
  Top 1.016: U$8.7 U$8.8 STRIPE5.3
S5_2  (via drill 0.6)
  Top 0.406: IC1.33 42.63,41.36 43.18,41.91 46.35,41.91 v46.35,41.27 | v23.81,55.88 22.33,55.88 R32.1
  Bottom 0.406: v46.35,41.27 45.72,41.91 44.45,41.91 41.27,45.09 26.67,45.09 26.04,45.72 26.04,52.7 24.77,53.98 24.77,54.93 v23.81,55.88
S5_2O
  Top 1.016: U$7.6 U$7.5 STRIPE5.2
S5_3  (via drill 0.6)
  Top 0.406: IC1.32 44.48,40.03 v45.09,40.64 | v24.45,52.39 22.44,52.39 R31.1
  Bottom 0.406: v45.09,40.64 44.45,41.27 43.81,41.27 40.96,44.13 26.04,44.13 25.08,45.09 25.08,51.75 v24.45,52.39
S5_3O
  Top 1.016: U$7.8 U$7.7 STRIPE5.1
S6_1  (via drill 0.6)
  Top 0.406: v47.62,35.56 46.99,35.56 46.35,36.2 45.72,36.2 45.09,36.83 IC1.28 | R34.1 23.81,61.28 v25.72,59.37
  Bottom 0.406: v47.62,35.56 48.26,36.2 48.26,43.18 45.72,43.18 41.27,47.62 27.3,47.62 26.99,47.94 26.99,53.02 25.72,54.29 v25.72,59.37
S6_1O
  Top 1.016: U$8.6 U$8.5 7.62,62.23 STRIPE6.1
TX  (via drill 0.6)
  Top 0.406: IC1.17 36.83,27.94 32.38,23.5 32.38,19.68 31.91,19.21 | DATA.1 11.43,5.71 19.05,5.71 20.32,6.99 20.32,10.16 20.95,10.79 25.4,10.79 26.67,12.06 26.67,13.34 | 26.67,13.34 26.67,14.61 27.94,15.88 28.57,15.88 31.91,19.21 | IC4.11 43.81,8.26 43.18,8.89 41.27,8.89 40.64,9.53 v40.64,10.16 | v27.3,13.34 26.67,13.34 | JP2.10 54.61,17.78 53.66,18.73 32.38,18.73 31.91,19.21
  Bottom 0.406: v27.3,13.34 27.94,13.34 31.11,10.16 v40.64,10.16

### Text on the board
tNames: Thalhammer Development / http://www.dothal.de | EasyRGB v1.0 | 1 | 1 | 1 | + -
